PROGRAM Communication
VAR
	fbKL6831KL6841Communication		: FB_KL6831KL6841Communication;
	fbKL6831KL6841Config			: FB_KL6831KL6841Config;
	stInData			 			: ST_KL6831KL6841InData;
	stOutData		 	 			: ST_KL6831KL6841OutData;
	bConfigurate					: BOOL;	
END_VAR

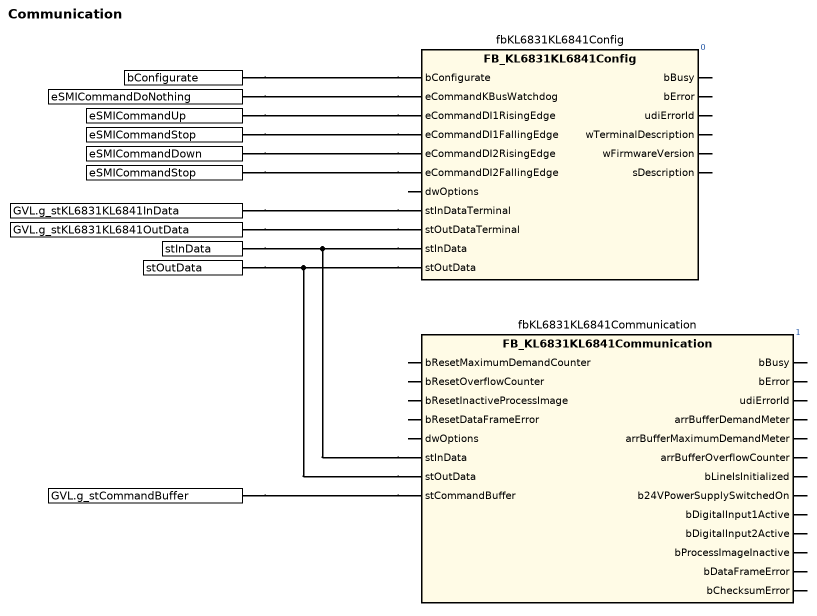
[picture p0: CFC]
fbKL6831KL6841Config(
    bConfigurate := bConfigurate,
    eCommandKBusWatchdog := eSMICommandDoNothing,
    eCommandDI1RisingEdge := eSMICommandUp,
    eCommandDI1FallingEdge := eSMICommandStop,
    eCommandDI2RisingEdge := eSMICommandDown,
    eCommandDI2FallingEdge := eSMICommandStop,
    stInDataTerminal := GVL.g_stKL6831KL6841InData,
    stOutDataTerminal := GVL.g_stKL6831KL6841OutData,
    stInData := stInData,
    stOutData := stOutData); // FB_KL6831KL6841Config
fbKL6831KL6841Communication(
    stInData := stInData,
    stOutData := stOutData,
    stCommandBuffer := GVL.g_stCommandBuffer); // FB_KL6831KL6841Communication

END_PROGRAM
